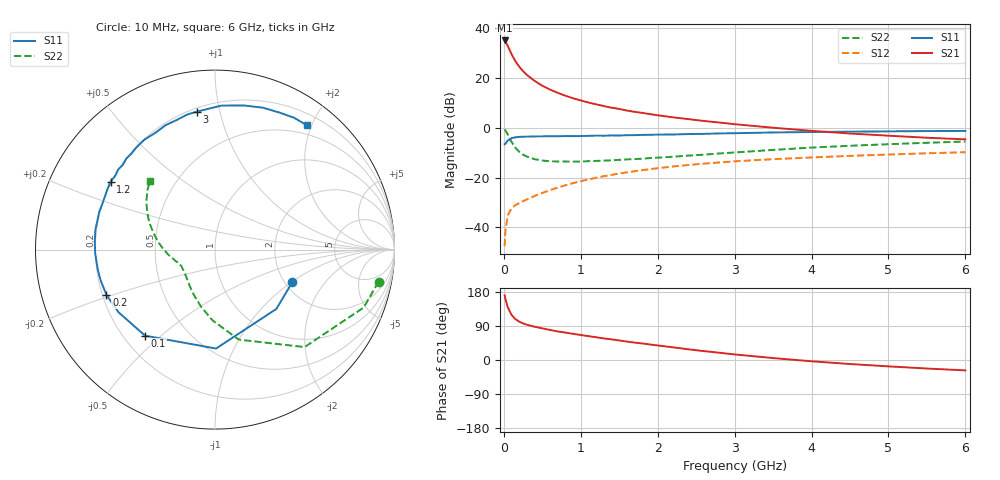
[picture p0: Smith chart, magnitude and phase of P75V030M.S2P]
! SIEMENS Small Signal Semiconductors
! BFP196
! Si NPN RF Bipolar Junction Transistor in SOT143
! VCE = 5 V  IC = 30 mA
! Common Emitter S-Parameters:  May  1996
# GHz  S  MA  R  50
!  f  S11  S21  S12  S22
! GHz  MAG  ANG  MAG  ANG  MAG  ANG  MAG  ANG
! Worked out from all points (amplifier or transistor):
!   36 points, 10 MHz to 6 GHz, reference 50 ohm
!   highest |S21| = 35.0 dB at 10 MHz (marker M1)
!   |S21| within 3 dB of that: start of sweep to 63.15 MHz
!   unconditionally stable (mu >= 1): 593.5 MHz to 3.941 GHz
!   at 250 MHz: K = 0.70, MSG = 26.1 dB, |S12| = -29.5 dB
!   at 1.4 GHz: K = 1.09, MAG = 11.6 dB, |S12| = -18.9 dB
!   at 6 GHz: K = 0.96, MSG = 2.6 dB, |S12| = -9.8 dB
!   lowest NFmin = 1.40 dB at 500 MHz
!   S11 on the Smith chart (normalised r, x): 10 MHz: 2.18, -1.02; 100 MHz: 0.29, -0.44; 200 MHz: 0.22, -0.19; 1.2 GHz: 0.20, +0.29; 3 GHz: 0.22, +0.85; 6 GHz: 0.36, +1.93
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0.01  0.4669 -23.0  56.35 170.9  0.0042 83.1  0.9287 -11.1
0.02  0.4756 -44.0  53.74 161.0  0.0084 73.8  0.8891 -21.3
0.05  0.5512 -89.4  44.19 139.7  0.0172 58.9  0.7378 -47.4
0.1  0.6179 -129.1  29.94 118.9  0.0242 47.6  0.5186 -75.2
0.15  0.641 -147.0  21.66 107.9  0.0281 44.3  0.3956 -91.8
0.2  0.6554 -157.3  16.83 101.2  0.0307 45.1  0.3291 -103.4
0.25  0.6599 -164.9  13.58 96.5  0.0336 46.3  0.2871 -112.6
0.3  0.6624 -170.5  11.45 93.1  0.0364 48.0  0.264 -119.4
0.4  0.668 -178.3  8.697 87.8  0.0427 51.5  0.2337 -130.0
0.5  0.6714 176.0  6.966 83.5  0.0491 54.1  0.2192 -137.6
0.6  0.6754 170.7  5.825 79.3  0.0558 55.4  0.2128 -142.8
0.7  0.675 166.0  5.013 75.4  0.063 56.8  0.21 -146.8
0.9  0.6773 158.0  3.9 69.1  0.0774 57.0  0.2083 -152.9
1.1  0.6873 150.8  3.205 62.9  0.0919 56.4  0.213 -156.8
1.2  0.6943 146.9  2.947 60.0  0.0989 55.9  0.2157 -158.7
1.6  0.7083 134.1  2.21 48.6  0.1272 51.9  0.2315 -165.0
2.2  0.7307 117.1  1.616 33.4  0.1668 44.5  0.2619 -173.9
3  0.7755 97.4  1.178 14.7  0.2116 33.8  0.3187 172.5
3.5  0.8032 87.4  0.999 5.1  0.2337 27.2  0.3586 164.3
4.5  0.8347 71.3  0.765 -10.6  0.2722 15.7  0.4341 150.6
5.5  0.8568 59.0  0.629 -22.5  0.3068 5.0  0.4989 139.1
6  0.8615 53.4  0.584 -27.4  0.3226 -0.8  0.528 133.5
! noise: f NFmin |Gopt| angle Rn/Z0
0.5  1.4  0.4  -173  0.08
0.9  1.6  0.5  -166  0.08
1.5  2.4  0.61  -150  0.14
2  2.9  0.71  -129  0.2
